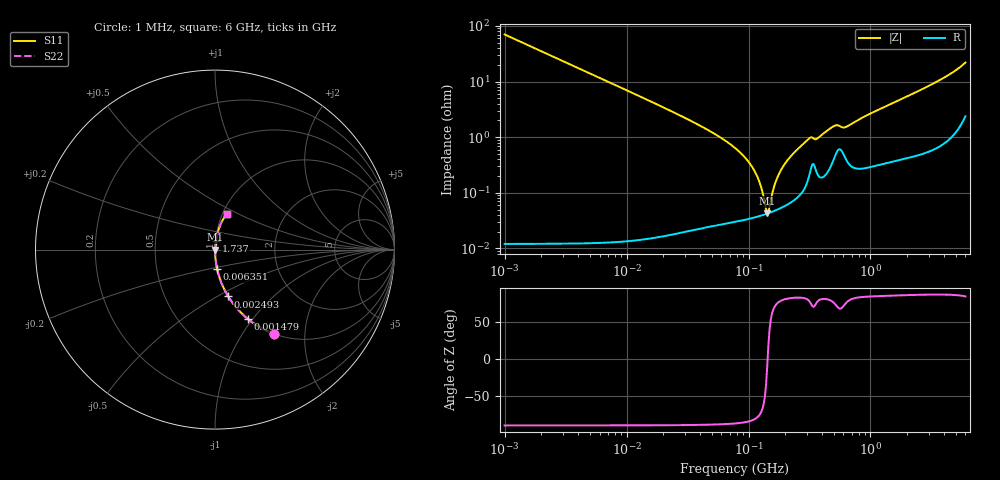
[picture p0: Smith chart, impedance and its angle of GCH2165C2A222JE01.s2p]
!Murata Part Number: GCH2165C2A222JE01
!These Parameters are Measured in Series Mode Connection
!Data Generated on Jun 19, 2026
!  o--ll--o
!Port1  Port2
!  o------o
!Operation Temp=25[degC], DC Bias Voltage=0[V]
!Freq. Start=1000[kHz] Stop=6[GHz] 401[Steps]
# Hz S RI R 50
!Freq.(Hz) S11(Real) S11(Imag) S21(Real) S21(Imag) S12(Real) S12(Imag) S22(Real) S22(Imag)
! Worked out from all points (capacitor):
!   401 points, 1 MHz to 6 GHz, reference 50 ohm
!   read as one part in series: C = 2.27 nF near 1.044 MHz
!   lowest |Z| = 42.9 mohm at 142.4 MHz (marker M1)
!   series resonance near 143.4 MHz, so ESL is about 540 pH
!   S11 on the Smith chart (normalised r, x): 1 MHz: 1.00, -1.40; 1.479 MHz: 1.00, -0.95; 2.493 MHz: 1.00, -0.56; 6.351 MHz: 1.00, -0.22; 1.737 GHz: 1.01, +0.09; 6 GHz: 1.05, +0.44
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1000000  0.3304 -0.4703  0.6696 0.4703  0.6696 0.4703  0.3304 -0.4703
1479166  0.1841 -0.3874  0.8159 0.3874  0.8159 0.3874  0.1841 -0.3874
2492906  0.0736 -0.2609  0.9264 0.2609  0.9264 0.2609  0.0736 -0.2609
4293785  0.0261 -0.1592  0.9739 0.1592  0.9739 0.1592  0.0261 -0.1592
6351220  0.0122 -0.109  0.9878 0.109  0.9878 0.109  0.0122 -0.109
1.843659e7  0.00156 -0.0374  0.9984 0.0374  0.9984 0.0374  0.00156 -0.0374
4.596069e7  0.000427 -0.0136  0.9996 0.0136  0.9996 0.0136  0.000427 -0.0136
7.745967e7  0.000341 -0.00639  0.9997 0.00639  0.9997 0.00639  0.000341 -0.00639
1.121107e8  0.000366 -0.00243  0.9996 0.00243  0.9996 0.00243  0.000366 -0.00243
1.249896e8  0.000387 -0.00135  0.9996 0.00135  0.9996 0.00135  0.000387 -0.00135
1.424119e8  0.000423 -7.04e-05  0.9996 7.04e-05  0.9996 7.04e-05  0.000423 -7.04e-05
1.487431e8  0.000437 0.000355  0.9996 -0.000355  0.9996 -0.000355  0.000437 0.000355
1.694764e8  0.000493 0.00165  0.9995 -0.00165  0.9995 -0.00165  0.000493 0.00165
1.930997e8  0.000569 0.00298  0.9994 -0.00298  0.9994 -0.00298  0.000569 0.00298
2.506837e8  0.00085 0.00592  0.9992 -0.00592  0.9992 -0.00592  0.00085 0.00592
3.325952e8  0.00328 0.00931  0.9967 -0.00931  0.9967 -0.00931  0.00328 0.00931
3.708027e8  0.00216 0.00938  0.9978 -0.00938  0.9978 -0.00938  0.00216 0.00938
5.138348e8  0.00489 0.0154  0.9951 -0.0154  0.9951 -0.0154  0.00489 0.0154
6.386712e8  0.00397 0.0149  0.996 -0.0149  0.996 -0.0149  0.00397 0.0149
1.428092e9  0.00496 0.038  0.995 -0.038  0.995 -0.038  0.00496 0.038
1.73686e9  0.00604 0.0463  0.994 -0.0463  0.994 -0.0463  0.00604 0.0463
6e9  0.0658 0.1995  0.9342 -0.1995  0.9342 -0.1995  0.0658 0.1995
